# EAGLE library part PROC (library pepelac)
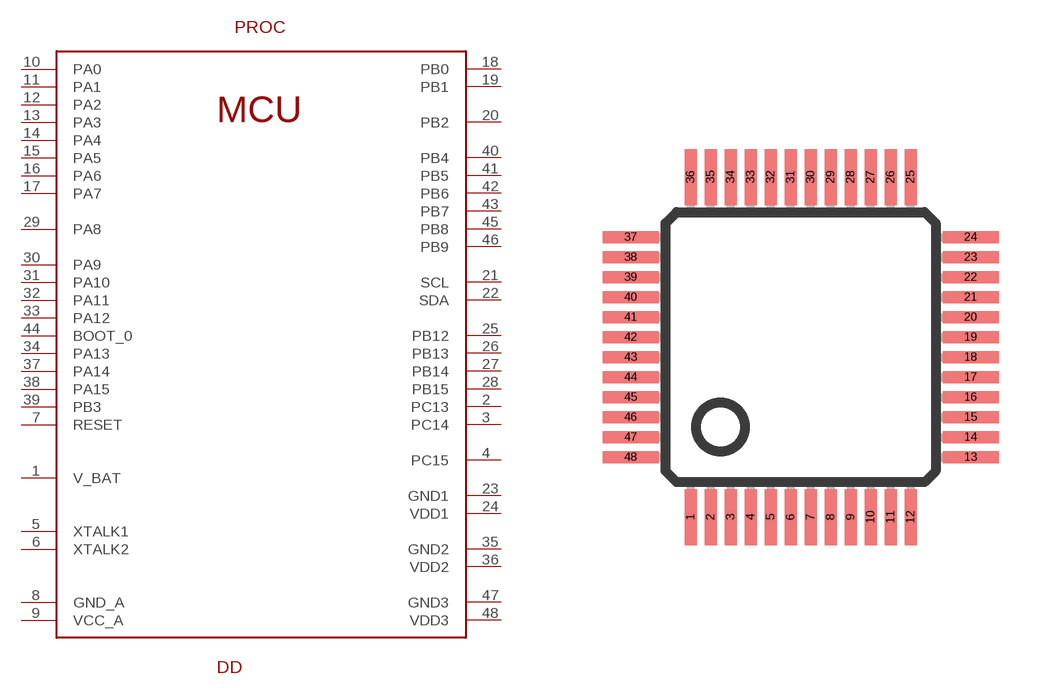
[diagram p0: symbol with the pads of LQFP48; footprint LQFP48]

Designator prefix DD

## PROC  [LQFP48]
1  V_BAT
2  PC13
3  PC14
4  PC15
5  XTALK1
6  XTALK2
7  RESET
8  GND_A
9  VCC_A
10  PA0
11  PA1
12  PA2
13  PA3
14  PA4
15  PA5
16  PA6
17  PA7
18  PB0
19  PB1
20  PB2
21  SCL
22  SDA
23  GND1
24  VDD1
25  PB12
26  PB13
27  PB14
28  PB15
29  PA8
30  PA9
31  PA10
32  PA11
33  PA12
34  PA13
35  GND2
36  VDD2
37  PA14
38  PA15
39  PB3
40  PB4
41  PB5
42  PB6
43  PB7
44  BOOT_0
45  PB8
46  PB9
47  GND3
48  VDD3

## Footprint LQFP48 (pad centres in mm)
48-pin plastic LQFP (FPT-48P-M26) www.fma.fujitsu.com/pdf/e713717.pdf
smd 0.3 x 1.4: 1 -2.75,-4.25; 2 -2.25,-4.25; 3 -1.75,-4.25; 4 -1.25,-4.25; 5 -0.75,-4.25; 6 -0.25,-4.25; 7 0.25,-4.25; 8 0.75,-4.25; 9 1.25,-4.25; 10 1.75,-4.25; 11 2.25,-4.25; 12 2.75,-4.25; 25 2.75,4.25; 26 2.25,4.25; 27 1.75,4.25; 28 1.25,4.25; 29 0.75,4.25; 30 0.25,4.25; 31 -0.25,4.25; 32 -0.75,4.25; 33 -1.25,4.25; 34 -1.75,4.25; 35 -2.25,4.25; 36 -2.75,4.25
smd 1.4 x 0.3: 13 4.25,-2.75; 14 4.25,-2.25; 15 4.25,-1.75; 16 4.25,-1.25; 17 4.25,-0.75; 18 4.25,-0.25; 19 4.25,0.25; 20 4.25,0.75; 21 4.25,1.25; 22 4.25,1.75; 23 4.25,2.25; 24 4.25,2.75; 37 -4.25,2.75; 38 -4.25,2.25; 39 -4.25,1.75; 40 -4.25,1.25; 41 -4.25,0.75; 42 -4.25,0.25; 43 -4.25,-0.25; 44 -4.25,-0.75; 45 -4.25,-1.25; 46 -4.25,-1.75; 47 -4.25,-2.25; 48 -4.25,-2.75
